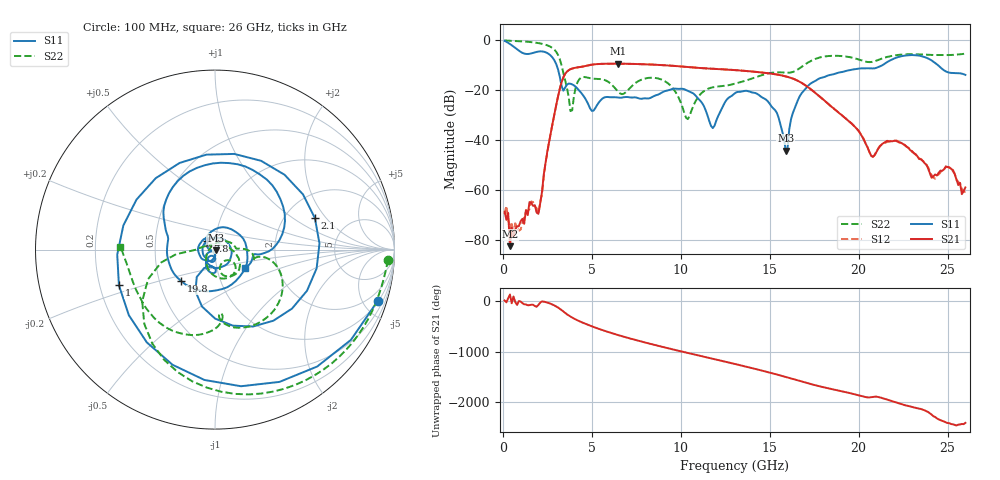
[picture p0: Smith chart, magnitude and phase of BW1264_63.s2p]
!Keysight Technologies,N5245B,MY57181159,A.13.60.06
!Date: Friday, December 18, 2020 23:55:20
!Correction: S11(Full 2 Port(1,2))
!S21(Full 2 Port(1,2))
!S12(Full 2 Port(1,2))
!S22(Full 2 Port(1,2))
!S2P File: Measurements: S11, S21, S12, S22:
# Hz S  dB  R 50
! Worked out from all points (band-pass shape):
!   260 points, 100 MHz to 26 GHz, reference 50 ohm
!   highest |S21| = -9.60 dB at 6.5 GHz (marker M1); lowest = -82.6 dB at 400 MHz (marker M2)
!   |S21| within 3 dB of the highest: 3.634 GHz to 13.81 GHz (10.18 GHz wide, 117 % of centre)
!   lowest |S11| = -44.4 dB at 15.9 GHz (marker M3), VSWR 1.01, Z = 50.5 - j0.372 ohm
!   |S11| at or under -10 dB: 3.012 GHz to 21.38 GHz (18.37 GHz wide, 151 % of centre); 24.42 GHz to end of sweep
!   |S22| runs from -31.8 to -0.3 dB; largest |S21 - S12| = 0.0006
!   S11 on the Smith chart (normalised r, x): 100 MHz: 1.06, -6.28; 1 GHz: 0.28, -0.17; 2.1 GHz: 2.90, +1.54; 7.8 GHz: 0.91, +0.09; 19.8 GHz: 0.65, -0.24; 26 GHz: 1.37, -0.30
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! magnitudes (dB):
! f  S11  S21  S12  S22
! 100 MHz  -0.4  -68.9  -69.8  -0.3
! 300 MHz  -1.3  -69.3  -71.7  -0.4
! 400 MHz  -1.7  -82.6  -75.9  -0.4
! 1 GHz  -4.9  -72.7  -76.0  -0.6
! 2.1 GHz  -4.7  -65.5  -65.0  -1.5
! 3.3 GHz  -18.5  -17.1  -17.1  -10.2
! 3.8 GHz  -17.6  -11.8  -11.8  -28.6
! 4.5 GHz  -22.2  -10.7  -10.7  -14.9
! 6.5 GHz  -23.2  -9.6  -9.6  -21.0
! 7.8 GHz  -23.6  -9.8  -9.8  -16.0
! 8.8 GHz  -21.7  -10.1  -10.1  -15.7
! 10.4 GHz  -20.5  -11.0  -10.9  -31.8
! 11.8 GHz  -35.4  -11.6  -11.6  -19.0
! 13.1 GHz  -21.2  -12.2  -12.2  -17.5
! 14.9 GHz  -24.7  -13.4  -13.4  -13.5
! 15.9 GHz  -44.4  -14.7  -14.7  -13.2
! 16.4 GHz  -27.5  -15.8  -15.8  -12.6
! 17.4 GHz  -17.1  -20.4  -20.3  -8.2
! 19.8 GHz  -11.8  -35.0  -34.9  -7.5
! 20.8 GHz  -11.5  -46.9  -46.9  -8.8
! 21.7 GHz  -8.6  -40.7  -40.7  -6.7
! 26 GHz  -14.1  -59.1  -60.9  -5.6
